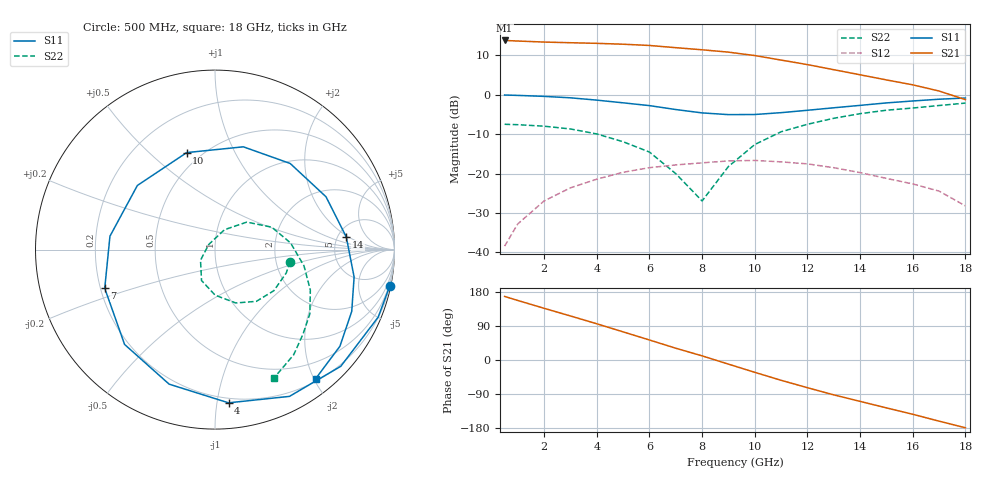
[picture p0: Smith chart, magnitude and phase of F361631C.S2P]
!ATF-36163
!1.5V 20mA
! last updated 11-10-95
# ghz s ma r 50
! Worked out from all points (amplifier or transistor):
!   19 points, 500 MHz to 18 GHz, reference 50 ohm
!   highest |S21| = 13.8 dB at 500 MHz (marker M1)
!   |S21| within 3 dB of that: start of sweep to 9.037 GHz
!   unconditionally stable (mu >= 1): 10.39 GHz to end of sweep
!   at 3 GHz: K = 0.37, MSG = 18.4 dB, |S12| = -23.6 dB
!   at 9 GHz: K = 0.92, MSG = 13.8 dB, |S12| = -16.8 dB
!   at 18 GHz: K = 1.56, MAG = 9.1 dB, |S12| = -28.2 dB
!   lowest NFmin = 0.51 dB at 2 GHz
!   S11 on the Smith chart (normalised r, x): 500 MHz: 0.24, -9.82; 4 GHz: 0.17, -1.08; 7 GHz: 0.22, -0.16; 10 GHz: 0.42, +0.66; 14 GHz: 5.98, +1.82; 18 GHz: 0.24, -2.03
0.5  0.995 -11.6  4.902 167.7  0.012 79.2  0.423 -9.3
1  0.984 -22.5  4.82 157.1  0.023 71.6  0.418 -18.0
2  0.956 -42.8  4.678 136.5  0.045 56.3  0.4 -34.9
3  0.917 -63.1  4.587 116.2  0.066 41.0  0.369 -51.4
4  0.857 -85.0  4.505 95.6  0.085 24.7  0.319 -68.7
5  0.792 -108.8  4.392 74.3  0.104 7.7  0.254 -89.8
6  0.73 -133.6  4.234 52.8  0.119 -9.1  0.188 -113.5
7  0.651 -160.7  3.97 31.1  0.129 -26.7  0.1 -143.8
8  0.59 172.7  3.732 10.9  0.137 -40.0  0.045 140.3
9  0.561 140.4  3.483 -10.9  0.145 -55.1  0.123 64.4
10  0.563 106.3  3.154 -32.5  0.147 -70.7  0.234 40.9
11  0.594 74.6  2.763 -53.5  0.141 -85.5  0.34 21.6
12  0.637 48.9  2.421 -73.1  0.133 -98.6  0.423 5.0
13  0.685 25.4  2.086 -92.0  0.119 -111.5  0.504 -10.3
14  0.735 5.5  1.798 -109.1  0.103 -120.8  0.577 -23.0
15  0.79 -11.2  1.547 -126.4  0.087 -129.9  0.638 -34.0
16  0.836 -24.3  1.34 -143.2  0.074 -136.4  0.68 -43.9
17  0.88 -37.7  1.118 -161.4  0.06 -144.5  0.732 -53.2
18  0.912 -52.0  0.87 -178.9  0.039 -151.5  0.786 -65.1
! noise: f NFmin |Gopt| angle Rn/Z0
2  0.51  0.864  28.49  0.397
3  0.55  0.755  42.63  0.329
5  0.65  0.593  73.26  0.202
7  0.75  0.466  107.4  0.115
9  0.87  0.301  143.9  0.076
10  0.94  0.219  178.7  0.076
12  1.11  0.223  -79.11  0.156
14  1.33  0.4  -12.95  0.377
16  1.62  0.608  20.88  0.71
18  2.04  0.714  51.57  1.315
